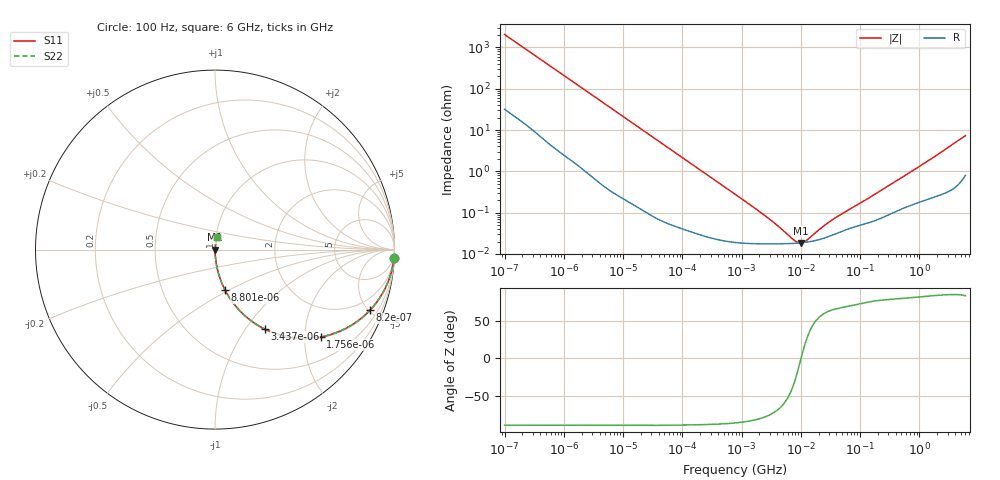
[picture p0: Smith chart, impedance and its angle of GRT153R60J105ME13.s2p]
!Murata Part Number: GRT153R60J105ME13
!These Parameters are Measured in Series Mode Connection
!Data Generated on Jun 19, 2026
!  o--ll--o
!Port1  Port2
!  o------o
!Operation Temp=25[degC], DC Bias Voltage=0[V]
!Freq. Start=100[Hz] Stop=6[GHz] 401[Steps]
# Hz S RI R 50
!Freq.(Hz) S11(Real) S11(Imag) S21(Real) S21(Imag) S12(Real) S12(Imag) S22(Real) S22(Imag)
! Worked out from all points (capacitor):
!   401 points, 100 Hz to 6 GHz, reference 50 ohm
!   read as one part in series: C = 773 nF near 109 Hz
!   lowest |Z| = 18.6 mohm at 9.942 MHz (marker M1)
!   series resonance near 10.08 MHz, so ESL is about 320 pH
!   S11 on the Smith chart (normalised r, x): 100 Hz: 2, -41; 820 Hz: 1.06, -5.10; 1.756 kHz: 1.03, -2.40; 3.437 kHz: 1.01, -1.23; 8.801 kHz: 1.00, -0.48; 6 GHz: 1.02, +0.15
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100  0.9969 -0.0485  0.00312 0.0485  0.00312 0.0485  0.9969 -0.0485
293  0.9786 -0.1378  0.0214 0.1378  0.0214 0.1378  0.9786 -0.1378
524  0.938 -0.2349  0.062 0.2349  0.062 0.2349  0.938 -0.2349
820  0.8639 -0.337  0.1361 0.337  0.1361 0.337  0.8639 -0.337
1174  0.7591 -0.4218  0.2409 0.4218  0.2409 0.4218  0.7591 -0.4218
1756  0.5886 -0.4864  0.4114 0.4864  0.4114 0.4864  0.5886 -0.4864
2008  0.5236 -0.4939  0.4764 0.4939  0.4764 0.4939  0.5236 -0.4939
3437  0.2765 -0.4422  0.7235 0.4422  0.7235 0.4422  0.2765 -0.4422
5378  0.1368 -0.3388  0.8632 0.3388  0.8632 0.3388  0.1368 -0.3388
8801  0.0571 -0.227  0.9429 0.227  0.9429 0.227  0.0571 -0.227
18016  0.0151 -0.1165  0.9849 0.1165  0.9849 0.1165  0.0151 -0.1165
40335  0.00349 -0.0529  0.9965 0.0529  0.9965 0.0529  0.00349 -0.0529
774597  0.000198 -0.00281  0.9998 0.00281  0.9998 0.00281  0.000198 -0.00281
2967816  0.000176 -0.000674  0.9998 0.000674  0.9998 0.000674  0.000176 -0.000674
7599586  0.000181 -0.000124  0.9998 0.000124  0.9998 0.000124  0.000181 -0.000124
9941735  0.000186 -5.9e-06  0.9998 5.9e-06  0.9998 5.9e-06  0.000186 -5.9e-06
1.189169e7  0.000191 7.11e-05  0.9998 -7.11e-05  0.9998 -7.11e-05  0.000191 7.11e-05
1.555665e7  0.000204 0.00019  0.9998 -0.00019  0.9998 -0.00019  0.000204 0.00019
3.64232e7  0.000297 0.00065  0.9997 -0.00065  0.9997 -0.00065  0.000297 0.00065
3.124326e8  0.000924 0.00453  0.9991 -0.00453  0.9991 -0.00453  0.000924 0.00453
1.873145e9  0.00297 0.0233  0.997 -0.0233  0.997 -0.0233  0.00297 0.0233
6e9  0.013 0.0712  0.987 -0.0712  0.987 -0.0712  0.013 0.0712
